FUNCTION_BLOCK Example36_SetDateAndTime	//any combination of xbots and flyways - SetDateAndTime
VAR_INPUT
	Execute : BOOL;
END_VAR
VAR_OUTPUT
	Done : BOOL;
END_VAR
VAR_IN_OUT
	PM_Controller : PMControllerType;
END_VAR
VAR
	GetTime : NT_GetTime;
	PMC_SetDateAndTime1 : PMC_SetDateAndTime;
END_VAR

//any combination of xbots and flyways - SetDateAndTime

//get the PLC local time
GetTime(START := Execute);

//send the PLC local time to the PMC 
PMC_SetDateAndTime1(Execute := GetTime.START AND NOT(GetTime.BUSY) AND NOT(GetTime.ERR),Year := GetTime.TIMESTR.wYear,Month := GetTime.TIMESTR.wMonth,Day := GetTime.TIMESTR.wDay,Hour := GetTime.TIMESTR.wHour,Minute := GetTime.TIMESTR.wMinute,Second := GetTime.TIMESTR.wSecond,PM_Controller := PM_Controller);
Done := PMC_SetDateAndTime1.Done;

END_FUNCTION_BLOCK
